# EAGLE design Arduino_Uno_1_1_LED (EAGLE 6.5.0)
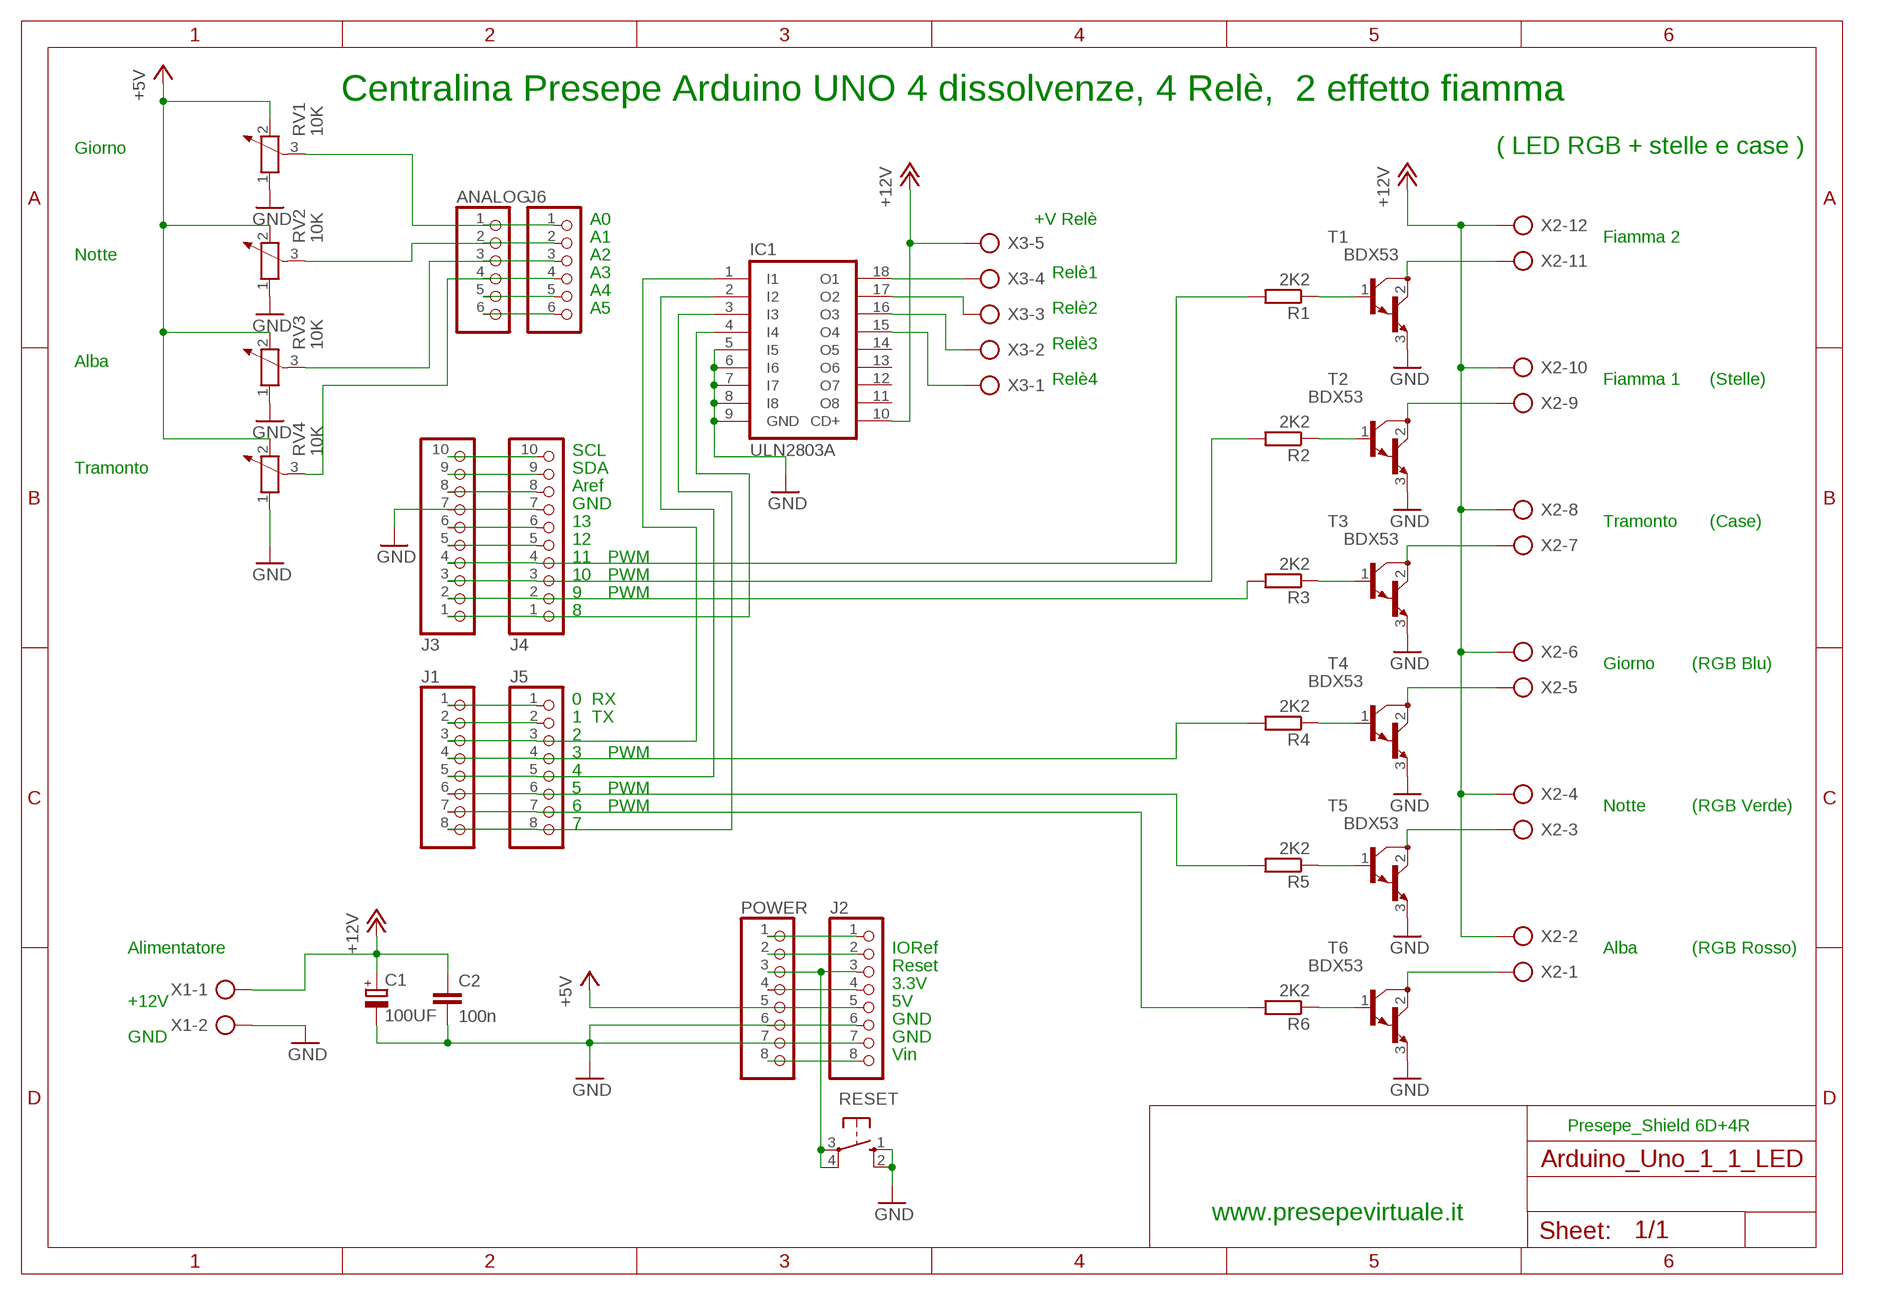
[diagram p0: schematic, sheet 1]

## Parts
ANALOG  PINHD-1X6  [1X06]
C1  100UF  CPOL-EUE5-4  [E5-4]
C2  100n  C-EU050-024X044  [C050-024X044]
IC1  ULN2803A  [DIL18]
J1  PINHD-1X8TH  [1X08-TH]
J2  PINHD-1X8TH  [1X08-TH]
J3  PINHD-1X10TH  [1X10-TH]
J4  PINHD-1X10TH  [1X10-TH]
J5  PINHD-1X8TH  [1X08-TH]
J6  PINHD-1X6  [1X06]
POWER  PINHD-1X8TH  [1X08-TH]
R1  2K2  R-EU_0207/5V  [0207/5V]
R2  2K2  R-EU_0207/5V  [0207/5V]
R3  2K2  R-EU_0207/5V  [0207/5V]
R4  2K2  R-EU_0207/5V  [0207/5V]
R5  2K2  R-EU_0207/5V  [0207/5V]
R6  2K2  R-EU_0207/5V  [0207/5V]
RESET  10-XX  [B3F-10XX]
RV1  10K  POTENTIOMETER_PT-10S  [PT-10S]
RV2  10K  POTENTIOMETER_PT-10S  [PT-10S]
RV3  10K  POTENTIOMETER_PT-10S  [PT-10S]
RV4  10K  POTENTIOMETER_PT-10S  [PT-10S]
T1  BDX53  [TO220]
T2  BDX53  [TO220]
T3  BDX53  [TO220]
T4  BDX53  [TO220]
T5  BDX53  [TO220]
T6  BDX53  [TO220]
X1  AK500/2  [AK500/2]
X2  AK500/12  [AK500/12]
X3  AK500/5  [AK500/5]

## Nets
+5V: J2.5 POWER.5 RV1.2 RV2.2 RV3.2 RV4.2
+9V: J2.8 POWER.8
+12V: C1.+ C2.1 IC1.10(CD+) X1.1 X2.2 X2.4 X2.6 X2.8 X2.10 X2.12 X3.5
GND: C1.- C2.2 IC1.5(I5) IC1.6(I6) IC1.7(I7) IC1.8(I8) IC1.9(GND) J2.6 J2.7 J3.7 J4.7 POWER.6 POWER.7 RESET.1(S) RESET.2(S1) RV1.1 RV2.1 RV3.1 RV4.1 T1.3(E) T2.3(E) T3.3(E) T4.3(E) T5.3(E) T6.3(E) X1.2
N$1: J3.5 J4.5
N$2: IC1.4(I4) J3.1 J4.1
N$3: J3.6 J4.6
N$4: R3.1 T3.1(B)
N$5: J3.4 J4.4 R1.2
N$6: J3.2 J4.2 R3.2
N$7: J3.3 J4.3 R2.2
N$8: J1.1 J5.1
N$9: J1.2 J5.2
N$10: IC1.1(I1) J1.3 J5.3
N$11: J1.4 J5.4 R4.2
N$12: R4.1 T4.1(B)
N$13: J1.6 J5.6 R5.2
N$14: J1.7 J5.7 R6.2
N$15: IC1.3(I3) J1.8 J5.8
N$16: T4.2(C) X2.5
N$17: R5.1 T5.1(B)
N$18: R6.1 T6.1(B)
N$19: ANALOG.2 J6.2 RV2.3
N$20: ANALOG.3 J6.3 RV3.3
N$21: ANALOG.4 J6.4 RV4.3
N$22: ANALOG.5 J6.5
N$23: ANALOG.6 J6.6
N$24: T6.2(C) X2.1
N$25: T5.2(C) X2.3
N$26: T3.2(C) X2.7
N$27: T1.2(C) X2.11
N$30: IC1.18(O1) X3.4
N$31: J2.2 POWER.2
N$32: J2.1 POWER.1
N$33: IC1.17(O2) X3.3
N$34: ANALOG.1 J6.1 RV1.3
N$43: IC1.16(O3) X3.2
N$44: IC1.15(O4) X3.1
N$49: R1.1 T1.1(B)
N$50: R2.1 T2.1(B)
N$52: T2.2(C) X2.9
N$54: IC1.2(I2) J1.5 J5.5
N$141: J3.9 J4.9
N$142: J3.10 J4.10
N$222: J3.8 J4.8
N$223: J2.4 POWER.4
RESET: J2.3 POWER.3 RESET.3(P) RESET.4(P1)
Unconnected: IC1.11(O8) IC1.12(O7) IC1.13(O6) IC1.14(O5)

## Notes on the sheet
- Centralina Presepe Arduino UNO 4 dissolvenze, 4 Relè,  2 effetto fiamma
- Giorno | ( LED RGB + stelle e case )
- A0 | +V Relè
- A1 | Fiamma 2
- Notte | A2
- A3 | Relè1
- A4
- A5 | Relè2
- Relè3
- Alba
- Relè4 | Fiamma 1 | (Stelle)
- SCL
- Tramonto | SDA
- Aref
- GND
- 13 | Tramonto | (Case)
- 12
- 11 | PWM
- 10 | PWM
- 9 | PWM
- 8
- Giorno | (RGB Blu)
- 0  RX
- 1  TX
- 2
- 3 | PWM
- 4
- 5 | PWM
- 6 | PWM | Notte | (RGB Verde)
- 7
- Alimentatore | IORef | Alba | (RGB Rosso)
- Reset
- 3.3V
- +12V | 5V
- GND
- GND | GND
- Vin
- Presepe_Shield 6D+4R
- www.presepevirtuale.it

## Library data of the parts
ANALOG J6 = pinhead:PINHD-1X6: PIN HEADER
C1 = rcl:CPOL-EU: POLARIZED CAPACITOR, European symbol
C2 = rcl:C-EU: CAPACITOR, European symbol
IC1 = uln-udn:ULN2803A: DRIVER ARRAY
J1 J2 J5 POWER = SmartPrj:PINHD-1X8: PIN HEADER
J3 J4 = SmartPrj:PINHD-1X10: PIN HEADER
R1-R6 = rcl:R-EU_: RESISTOR, European symbol
RESET = switch-omron:10-XX: OMRON SWITCH; MPN: B3F-1000; OC_FARNELL: 176432; OC_NEWARK: 36M3542
RV1-RV4 = rcl:POTENTIOMETER_: Potentiometer
T1-T6 = transistor:BDX53: NPN BIPOLAR DARLINGTON TRANSISTOR
X1 = con-ptr500:AK500/2: CONNECTOR; OC_FARNELL: unknown; OC_NEWARK: unknown
X2 = con-ptr500:AK500/12: CONNECTOR; OC_FARNELL: unknown; OC_NEWARK: unknown
X3 = con-ptr500:AK500/5: CONNECTOR; OC_FARNELL: unknown; OC_NEWARK: unknown

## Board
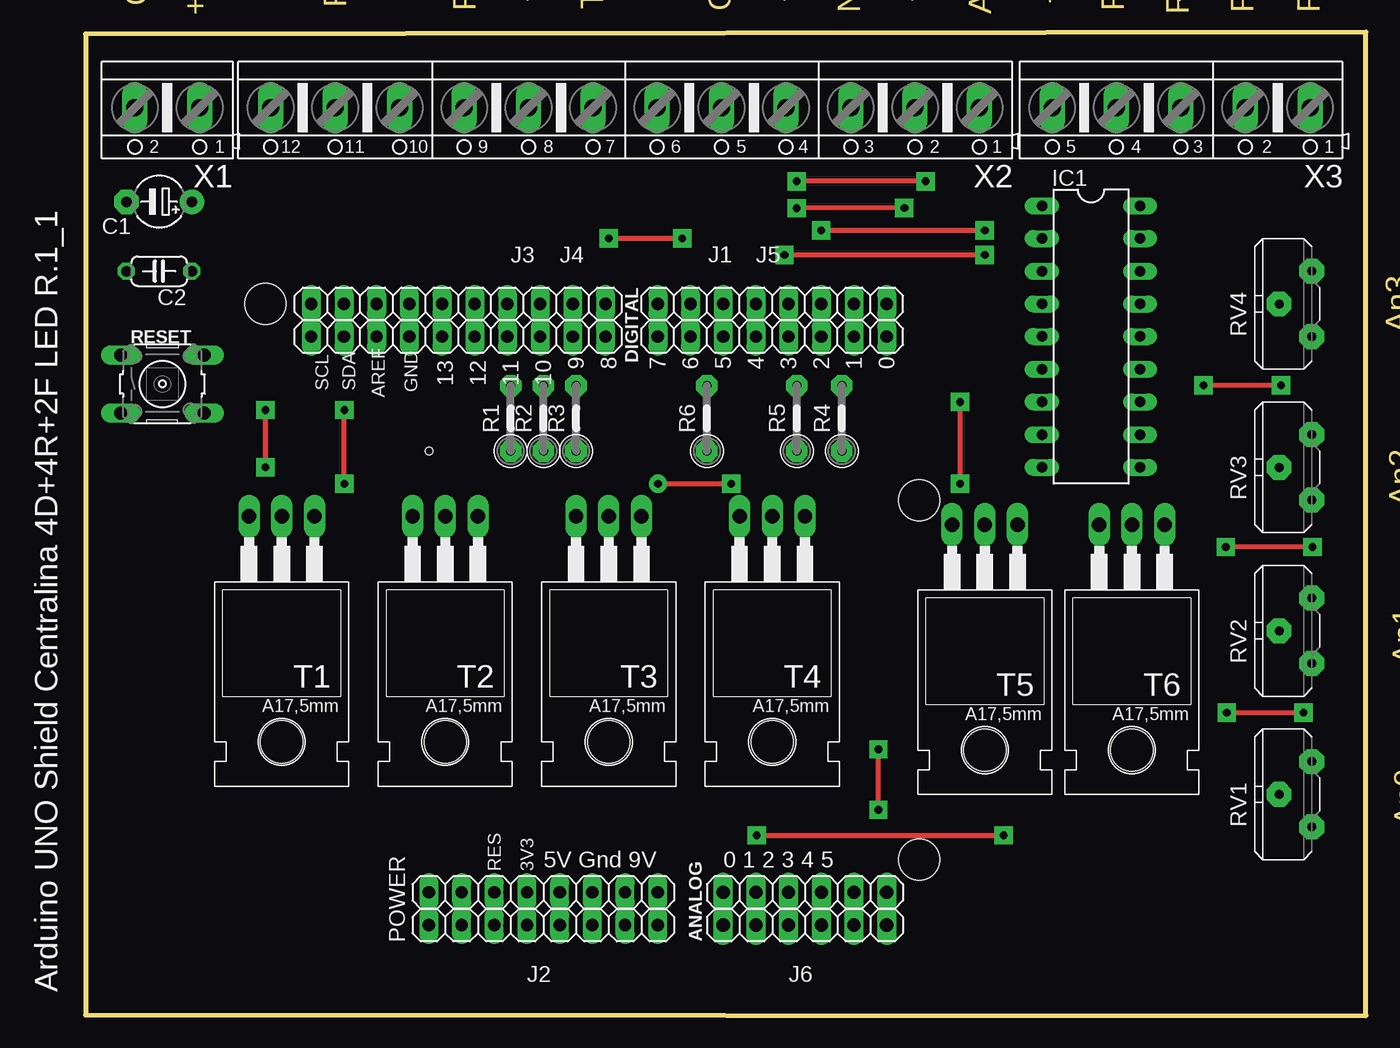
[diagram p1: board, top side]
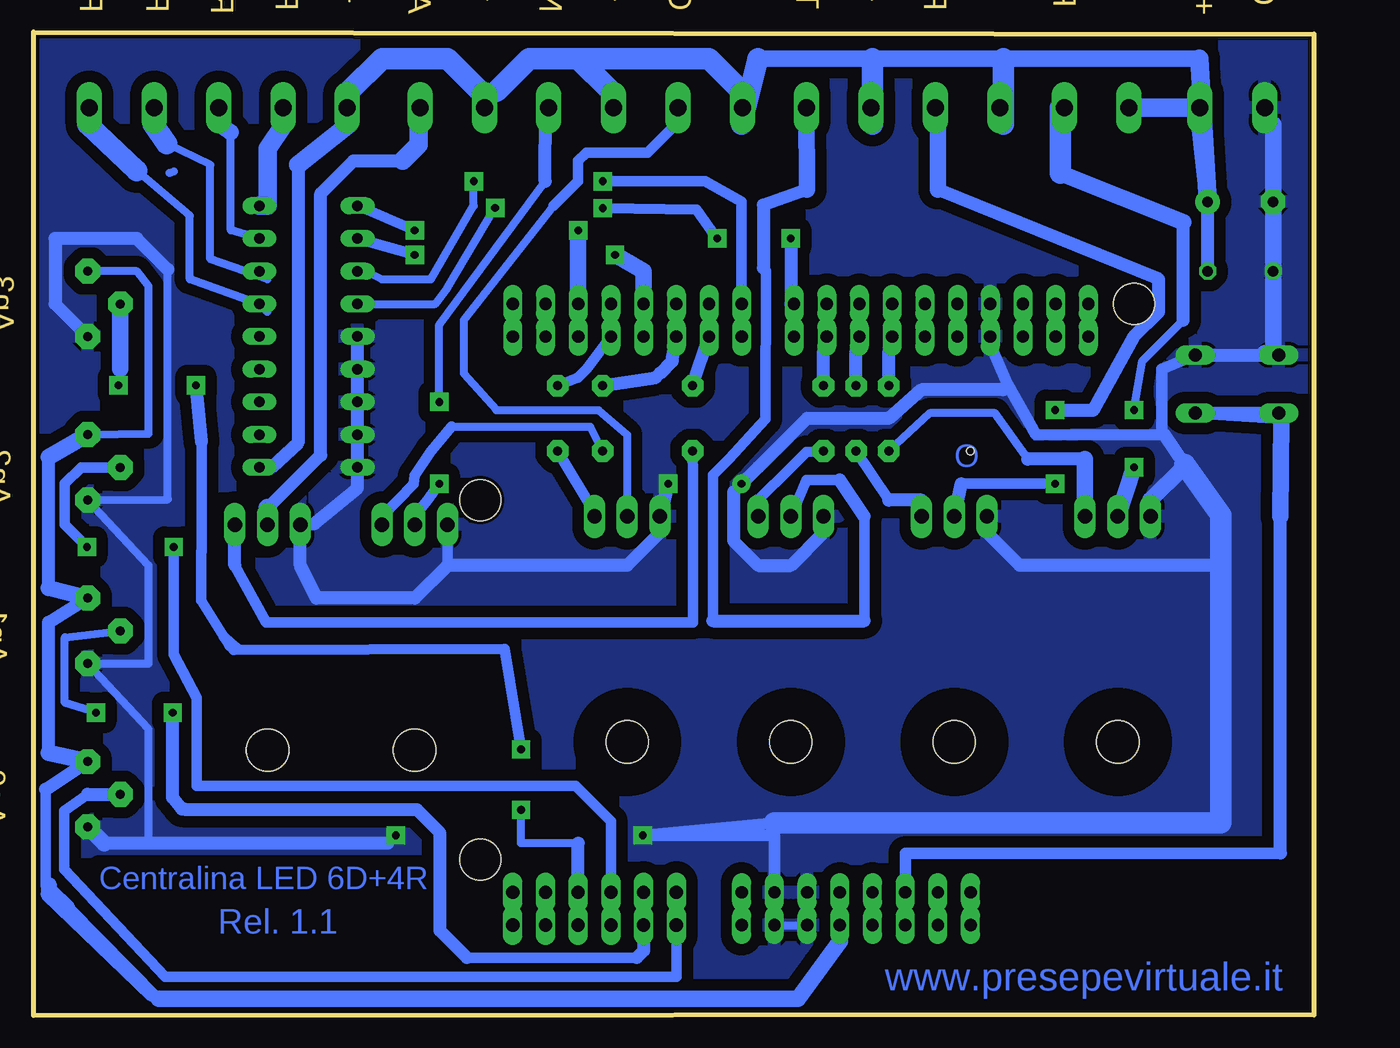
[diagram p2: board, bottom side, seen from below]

Size 99.46 x 76.4 mm. Coordinates in mm from the lower left corner, seen from the top.
Outline: 0,76.25 0,0.05 99.46,0 99.46,76.4 0,76.25
Copper layers (1*16): Top 0.035mm / dielectric 1.5mm / Bottom 0.035mm
Design rules "default *": minimum track width 24mil, minimum drill 20mil, track to track 35mil, track to pad 35mil, pad to pad 35mil, via to via 35mil, smd to smd 8mil, copper to edge 10mil, drill to drill 8mil, minimum pad ring 10mil, minimum via ring 8mil, stop-mask expansion 2mil, vias tented up to drill 0mil, thermal gap 10mil
Holes 3.2 mm at 13.97,55.29 64.77,12.11 64.77,40.05
Holes 0.6 mm at 26.67,43.86

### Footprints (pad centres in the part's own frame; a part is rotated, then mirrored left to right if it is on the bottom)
1X06 = drill 1.016 long: 1 -6.35,0; 2 -3.81,0; 3 -1.27,0; 4 1.27,0; 5 3.81,0; 6 6.35,0
E5-4 = drill 0.813 pad 1.905: + -2.54,0 | drill 0.813 pad 1.905 octagon: - 2.54,0
C050-024X044 = drill 0.813 octagon: 1 -2.54,0; 2 2.54,0
DIL18 = drill 0.813 long: 1 -10.16,-3.81; 2 -7.62,-3.81; 3 -5.08,-3.81; 4 -2.54,-3.81; 5 0,-3.81; 6 2.54,-3.81; 7 5.08,-3.81; 8 7.62,-3.81; 9 10.16,-3.81; 10 10.16,3.81; 11 7.62,3.81; 12 5.08,3.81; 13 2.54,3.81; 14 0,3.81; 15 -2.54,3.81; 16 -5.08,3.81; 17 -7.62,3.81; 18 -10.16,3.81
1X08-TH = drill 0.95 pad 1.422 long: 1 -8.89,0; 2 -6.35,0; 3 -3.81,0; 4 -1.27,0; 5 1.27,0; 6 3.81,0; 7 6.35,0; 8 8.89,0
1X10-TH = drill 0.95 pad 1.422 long: 1 -11.43,0; 2 -8.89,0; 3 -6.35,0; 4 -3.81,0; 5 -1.27,0; 6 1.27,0; 7 3.81,0; 8 6.35,0; 9 8.89,0; 10 11.43,0
0207/5V = drill 0.7 pad 1.676 octagon: 1 -2.54,0; 2 2.54,0
B3F-10XX = drill 1.016 long: 1 -3.251,2.261; 2 3.251,2.261; 3 -3.251,-2.261; 4 3.251,-2.261
PT-10S = drill 0.7 pad 1.93 octagon: 1 -2.54,-1.27; 2 2.54,-1.27; 3 0,1.27
TO220 = drill 1.118 long: 1 -2.54,-6.35; 2 0,-6.35; 3 2.54,-6.35 | hole 3.302: 0,11.176
AK500/2 = drill 1.321 long: 1 -2.515,0; 2 2.515,0
AK500/12 = drill 1.321 long: 1 -27.534,0; 2 -22.53,0; 3 -17.526,0; 4 -12.497,0; 5 -7.493,0; 6 -2.489,0; 7 2.489,0; 8 7.493,0; 9 12.497,0; 10 17.526,0; 11 22.53,0; 12 27.534,0
AK500/5 = drill 1.321 long: 1 -10.033,0; 2 -5.004,0; 3 0,0; 4 5.004,0; 5 10.008,0

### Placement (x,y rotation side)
ANALOG  55.88,7.03 0 top
C1  5.71,63.23 180 top
C2  5.71,57.83 180 top
IC1  78.11,52.75 270 top
J1  53.34,55.29 180 top
J2  35.56,7.03 0 top
J3  28.96,55.29 180 top
J4  28.96,52.75 180 top
J5  53.34,52.75 180 top
J6  55.88,9.57 0 top
POWER  35.56,9.57 0 top
R1  33.02,46.4 90 top
R2  35.56,46.4 90 top
R3  38.1,46.4 90 top
R4  58.74,46.4 90 top
R5  55.24,46.4 90 top
R6  48.26,46.4 90 top
RESET  5.97,49.07 0 top
RV1  93.98,17.19 90 top
RV2  93.98,29.89 90 top
RV3  93.98,42.59 90 top
RV4  93.98,55.29 90 top
T1  15.24,32.43 180 top
T2  27.94,32.43 180 top
T3  40.64,32.43 180 top
T4  53.34,32.43 180 top
T5  69.85,31.8 180 top
T6  81.28,31.8 180 top
X1  6.35,70.53 180 top
X2  41.91,70.53 180 top
X3  85.09,70.53 180 top

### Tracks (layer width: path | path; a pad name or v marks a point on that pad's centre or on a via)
+5V
  Bottom 0.61: POWER.5 J2.5 36.83,5.76 | RV4.2 91.44,57.83 90.52,56.65 90.52,45.22 RV3.2
  Bottom 0.813: 98.53,17.59 98.53,10.08 96.7,8.36 89.72,1.3
  Bottom 1.016: 98.53,17.59 RV1.2 | RV2.2 98.29,30.55 98.29,20.39 | 98.29,33.23 98.29,43.39 | 90.23,1.56 98.43,9.43 98.34,9.51 98.34,10.05 98.16,10.22 98.16,9.82 96.7,8.36
  Bottom 1.27: RV1.2 98.29,20.39 | 98.29,43.39 RV3.2 | RV2.2 98.29,33.23 | 36.83,5.76 40.06,1.3 89.72,1.3
+9V
  Bottom 0.61: J2.8 POWER.8
+12V
  Bottom 0.61: 24.13,69.26 X2.10 | 34.29,69.26 X2.8 | 44.45,69.26 X2.6 44.45,71.8 | 8.89,69.26 X1.1 | 54.61,71.8 X2.4 | 63.5,71.8 X2.2 64.77,71.8 | 80.96,42.59 IC1.10 | 74.93,69.26 X3.5 74.93,71.8
  Bottom 1.016: C2.1 C1.+ | 80.96,42.59 78.92,44.5 78.92,66.09
  Bottom 1.27: 8.89,74.34 24.13,74.34 34.29,74.34 43.18,74.34 | C1.+ 8.89,69.26
  Bottom 1.422: X1.1 X2.12 | C1.+ 8.89,74.34 | 74.93,69.26 78.92,66.09
  Bottom 1.676: 24.13,74.34 24.13,69.26 | 34.29,74.34 34.29,69.26 | 43.18,74.34 44.45,69.26 | 57.15,74.34 54.61,71.8 | 57.15,74.34 60.96,74.34 63.5,71.8 | 64.77,71.8 67.31,74.34 72.39,74.34 74.93,71.8 | 44.45,71.8 46.99,74.34 57.15,74.34
GND  (via drill 0.6 pad 1.42)
  Top 0.406: v52.14,14 v71.31,14 | v44.47,41.32 v50.16,41.32
  Bottom 0.406: 45.08,40.69 v44.47,41.32
  Bottom 0.61: J4.7 J3.7 | POWER.7 J2.7 J2.6 POWER.6 | 90.52,13.38 90.52,22.27 RV2.1 90.52,27.35 90.52,34.97 RV3.1 89.03,40.1 89.03,57.96 | 3.81,69.26 X1.2 | 12.7,40.05 T1.3 | 10.01,42.82 10.16,42.59 | 25.4,37.51 T2.3 | 44.09,41.69 45.08,40.69 | 23.82,49.07 24.13,48.63 | RESET.1 3.81,51.48 | v71.31,14 71.92,13.38
  Bottom 0.813: 67.31,34.97 T5.3
  Bottom 0.889: 41.91,14.99 v52.14,14 41.9,14 41.9,13.65 POWER.7 | RESET.2 11.8,50.21 11.8,45.13 11.59,45.12 21.59,45.13 23.82,49.07 25.4,52.75 J4.7
  Bottom 1.016: RESET.2 RESET.1 | 10.01,42.82 11.59,45.12 | 93.98,13.38 90.52,13.38 82.55,13.38 81.12,13.38 80.01,13.38 71.92,13.38 | 89.03,57.96 91.44,60.37 97.79,60.37 97.79,55.29 RV4.1 | IC1.5 IC1.6 IC1.7 IC1.8 IC1.9 74.3,41.01 77.66,38.21 T6.3 78.74,34.97 77.47,32.43 69.85,32.43 67.31,34.97 53.34,34.97 50.8,37.51 T4.3 v50.16,41.32 | 25.4,37.51 22.86,34.97 7.23,34.97 | 45.08,40.69 45.08,36.88 43.18,34.97 40.64,34.97 38.1,37.51 T3.3 | 44.09,41.69 43.18,42.59 39.37,46.4 33.02,46.4 30.48,48.63 24.13,48.63
  Bottom 1.27: 93.98,13.38 RV1.1 | 3.81,69.26 3.18,69.26 C1.- C2.2 3.18,51.48 3.81,51.48 | 10.16,42.59 12.7,40.05
  Bottom 1.676: 10.01,42.82 7.23,38.89 7.23,34.97 7.23,14.99 41.91,14.99
  pour Bottom: -0.32,76.25 99.7,76.25 99.7,-0.27 -0.32,-0.27
N$1
  Bottom 0.61: J4.5 J3.5
N$2  (via drill 0.6 pad 1.42)
  Top 0.406: v63.6,62.75 v55.24,62.72 | v46.35,60.37 v40.64,60.37
  Bottom 0.406: 40.64,55.29 J3.1
  Bottom 0.61: J4.1 J3.1 | IC1.4 68.26,55.29 67.31,56.56 v63.6,62.75
  Bottom 0.813: v55.24,62.72 47.94,62.59 v46.35,60.37
  Bottom 1.016: v40.64,60.37 40.64,55.29
N$3
  Bottom 0.61: J4.6 J3.6
N$4
  Bottom 0.813: R3.1 39.42,43.79 40.64,42.59 43.18,40.05
  Bottom 1.016: T3.1 43.18,40.05
N$5
  Bottom 0.61: J4.4 J3.4
  Bottom 1.016: R1.2 33.02,51.48 J4.4
N$6
  Bottom 0.61: J4.2 J3.2
  Bottom 1.016: R3.2 38.1,51.48 J4.2
N$7
  Bottom 0.61: J4.3 J3.3
  Bottom 1.016: R2.2 35.56,51.48 J4.3
N$8
  Bottom 0.61: J5.1 J1.1
N$9
  Bottom 0.61: J5.2 J1.2
N$10  (via drill 0.6 pad 1.42)
  Top 0.406: v57.15,61.01 v69.85,61.01
  Bottom 0.61: J5.3 J1.3
  Bottom 0.813: v69.85,61.01 IC1.1
  Bottom 1.27: J1.3 v57.15,61.01
N$11
  Bottom 0.61: J5.4 J1.4
  Bottom 0.813: R4.2 57.15,49.58 56.51,50.21 J5.4
N$12
  Bottom 0.813: 55.88,39.1 R4.1
  Bottom 1.016: T4.1 55.88,39.1
N$13
  Bottom 0.61: J5.6 J1.6 | 51.12,49.58 52.39,49.26 50.8,49.9
  Bottom 1.016: R5.2 51.12,49.58 | 50.8,49.9 49.85,50.85 J5.6
N$14
  Bottom 0.61: J5.7 J1.7
  Bottom 1.016: R6.2 J5.7
N$15  (via drill 0.6 pad 1.42)
  Top 0.406: v65.26,64.82 v55.24,64.82
  Bottom 0.61: J5.8 J1.8 | IC1.3 73.66,57.83 72.39,57.2 68.58,57.2 65.26,62.91 v65.26,64.82
  Bottom 0.813: v55.24,64.82 47.31,64.82 44.45,63.23 J1.8
N$16
  Bottom 0.61: 59.05,62.91 66.04,54.02 66.04,49.9 63.5,47.04 55.56,47.04 53.34,45.13 T4.2
  Bottom 0.813: 59.05,62.91 57.15,64.82 57.15,66.41 56.51,67.04 51.75,67.04 49.4,69.39 X2.5
N$17
  Bottom 0.61: R5.1 56.2,45.73 66.99,45.73 66.99,45.77 | 72.39,38.78 T5.1
  Bottom 0.813: 66.99,45.77 68.58,43.86 69.85,41.96 69.94,41.29 72.39,38.78
N$18
  Bottom 0.813: R6.1 48.22,41.91 48.23,30.54 81.38,30.54 83.82,34.97
  Bottom 1.016: 83.82,34.97 T6.1
N$19  (via drill 0.6 pad 1.42)
  Top 0.406: v88.65,23.54 v94.62,23.54
  Bottom 0.61: ANALOG.2 J6.2 | v94.62,23.54 97.02,24.31 97.02,29.39 RV2.3
  Bottom 0.813: 52.62,4.49 65.79,4.49
  Bottom 1.016: J6.2 52.07,5.04 52.62,4.49 | 65.79,4.49 67.88,6.59 67.88,14.19 69.68,15.99 87.64,15.99 87.7,16.05 87.94,16.05 88.67,16.95 88.67,23.48 v88.65,23.54
N$20  (via drill 0.6 pad 1.42)
  Top 0.406: v95.3,36.41 v88.58,36.41
  Bottom 0.61: ANALOG.3 J6.3
  Bottom 0.813: RV3.3 95.76,42.59 97.03,41.33 97.03,38.14 v95.3,36.41 | v88.58,36.41 88.58,28.04 86.77,24.68 86.77,17.86 57.36,17.86 54.6,15.1 J6.3
N$21  (via drill 0.6 pad 1.42)
  Top 0.406: v86.84,48.97 v92.86,48.97 | v61.58,15.98 v61.58,20.68
  Bottom 0.406: 86.38,45.33 86.41,44.59 | v92.86,48.97 92.71,50.21
  Bottom 0.61: ANALOG.4 J6.4 | 57.15,13.38 61.59,13.38 v61.58,15.98
  Bottom 0.813: v61.58,20.68 62.85,28.47 83.92,28.42 84.7,29.46 83.69,28.51 84.01,28.79 84.24,28.7 86.42,32.27 86.42,36.08 86.4,36.08 86.38,45.33
  Bottom 1.016: J6.4 57.15,13.38 | 86.41,44.59 v86.84,48.97
  Bottom 1.27: 92.71,50.21 RV4.3
N$22
  Bottom 0.61: ANALOG.5 J6.5
N$23
  Bottom 0.61: ANALOG.6 J6.6
N$24
  Bottom 1.016: 81.28,39.42 77.15,43.55 77.15,63.87 74.61,66.41 70.8,66.41
  Bottom 1.422: T6.2 81.28,39.42 | 70.8,66.41 69.53,67.67 69.53,70.44 X2.1
N$25  (via drill 0.6 pad 1.42)
  Top 0.406: v67.95,41.32 v67.95,47.67
  Bottom 0.406: 59.69,70.53 X2.3
  Bottom 0.61: v67.95,47.67 67.94,53.67 59.71,64.82
  Bottom 0.813: T5.2 69.85,38.78 68.73,40.2 v67.95,41.32
  Bottom 1.016: 59.71,64.82 59.69,70.53
N$26
  Bottom 0.61: 42.76,58.11 42.54,57.83
  Bottom 0.813: 42.54,57.83 42.6,46.34 45.42,43.23 46.68,41.99 46.68,30.67 | 34.92,30.66 34.92,38.78 | 36.83,41.62 39.43,41.62 T3.2
  Bottom 1.016: 39.37,64.18 42.76,62.97 42.76,58.11 | 46.68,30.67 34.92,30.66 | 34.92,38.78 36.83,41.62
  Bottom 1.27: X2.7 39.37,64.18
N$27  (via drill 0.6 pad 1.42)
  Top 0.406: v13.97,42.59 v13.97,47.04
  Bottom 0.406: 19.68,70.53 X2.11
  Bottom 0.61: v13.97,47.04 13.34,50.85 10.16,54.02
  Bottom 1.016: 10.16,54.02 10.16,61.64
  Bottom 1.27: T1.2 v13.97,42.59 | 10.16,61.64 19.68,65.45
  Bottom 1.676: 19.68,65.45 19.68,70.53
N$28
  Bottom 0.61: 88.9,65.45 88.55,65.57
N$30
  Bottom 0.61: 80.01,69.26 X3.4
  Bottom 1.422: IC1.18 81.28,62.91 81.28,67.36 80.01,69.26
N$31
  Bottom 0.61: J2.2 POWER.2
N$32
  Bottom 0.61: J2.1 POWER.1
N$33
  Bottom 0.61: 84.14,68.63 84.14,61.01 IC1.17 | 85.09,69.26 X3.3
  Bottom 1.27: 84.14,68.63 85.09,69.26
N$34
  Bottom 0.61: ANALOG.1 J6.1
  Bottom 0.813: J6.1 49.53,3.03 89.22,3.03 97.08,11.35 97.08,15.92 95.25,17.19
  Bottom 1.016: 95.25,17.19 RV1.3
N$43
  Bottom 0.61: 89.12,67.73 85.73,66.09 85.73,58.78 81.28,57.2 IC1.16
  Bottom 1.27: 90.17,69.26 X3.2
  Bottom 1.676: 89.12,67.73 90.17,69.26
N$44
  Bottom 0.61: 91.44,65.63 87.31,62.13 87.31,57.2 IC1.15 81.28,54.66 | 95.25,69.26 X3.1
  Bottom 1.676: 91.44,65.63 95.25,69.26
N$49
  Bottom 0.61: R1.1 29.84,46.8 24.77,46.8 22.23,43.23
  Bottom 1.016: 17.78,43.23 22.23,43.23
  Bottom 1.27: T1.1 17.78,43.23
N$50
  Bottom 0.813: 33.02,40.05 R2.1
  Bottom 1.016: 33.02,40.05 30.48,40.05 T2.1
N$52  (via drill 0.6 pad 1.42)
  Top 0.406: v20.1,41.32 v20.1,47.04
  Bottom 0.61: 29.21,70.53 X2.9
  Bottom 0.813: 27.39,41.32 v20.1,41.32
  Bottom 1.016: T2.2 27.39,41.32 | v20.1,47.04 17.14,47.04 13.97,52.75 12.07,54.66 12.07,57.2 29.21,64.18
  Bottom 1.27: 29.21,64.18 29.21,70.53 29.21,71.17
N$54  (via drill 0.6 pad 1.42)
  Top 0.406: v54.29,59.1 v69.85,59.1
  Bottom 0.61: J5.5 J1.5
  Bottom 0.813: v69.85,59.1 IC1.2
  Bottom 1.27: J1.5 52.07,57.83 v54.29,59.1
N$141
  Bottom 0.61: J4.9 J3.9
N$142
  Bottom 0.61: J4.10 J3.10
N$222
  Bottom 0.61: J4.8 J3.8
N$223
  Bottom 0.61: J2.4 POWER.4
RESET
  Bottom 0.61: POWER.3 J2.3
  Bottom 0.889: POWER.3 31.75,12.62 2.61,12.62 | 2.54,46.4 RESET.4
  Bottom 1.016: RESET.4 RESET.3 | 2.61,12.62 2.61,38.78
  Bottom 1.27: 2.61,38.78 2.54,46.4

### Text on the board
Bottom: O | Centralina LED 6D+4R | Rel. 1.1 | www.presepevirtuale.it
Dimension: +12V | +V | GND | Fiamma 2 | +V | Fiamma 1 (Stelle) | +V | Tramonto (Case) | +V | Giorno (RGB Blu) | +V | +V | +V | Relè 1 | Notte (RGB Verde) | Alba (RGB Rosso) | Relè 2 | Relè 3 | Relè 4 | An3 | An2 | An1 | An0
tPlace: 9 | 8 | 7 | 6 | 5 | 4 | 3 | 2 | 1 | 0 | 13 | 12 | 11 | 10 | Arduino UNO Shield Centralina 4D+4R+2F LED R.1_1
tNames: DIGITAL | AREF | SCL | SDA | GND | RES | 3V3 | 5V Gnd 9V | 0 1 2 3 4 5
bStop: DIGITAL | SDA | AREF | SCL | GND | 13 | 12 | 11 | 9 | 8 | 7 | 6 | 5 | 4 | 3 | 2 | 1 | 0 | 10 | 14 | 8 | 1 | 7 | 1 | 2 | 3 | 4 | +5V | GND | . | 5 | 6 | IOREF | RST | 3.3V | 5V | GND | GND | VIN | ANALOG | 0 | 1 | 2 | 3 | 4 | 5
Document: www.presepevirtuale.it
Reference: USB | ETH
